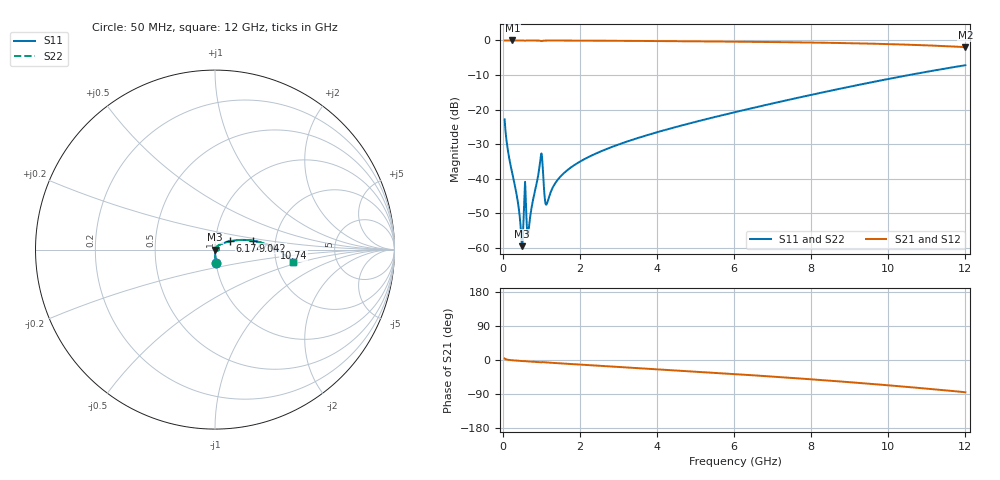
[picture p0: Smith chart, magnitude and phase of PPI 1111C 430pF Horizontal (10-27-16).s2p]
# MHz S MA R 50
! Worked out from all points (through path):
!   1601 points, 50 MHz to 12 GHz, reference 50 ohm
!   highest |S21| = 0.00 dB at 251.7 MHz (marker M1); lowest = -1.9 dB at 12 GHz (marker M2)
!   group delay of S21, straight-line fit = 19.3 ps
!   lowest |S11| = -59.5 dB at 505.6 MHz (marker M3), VSWR 1.00, Z = 50.1 - j0.027 ohm
!   |S11| at or under -10 dB: start of sweep to 10.54 GHz
!   |S22| runs from -59.5 to -7.2 dB; largest |S21 - S12| = 0
!   S11 on the Smith chart (normalised r, x): 50 MHz: 1.00, -0.14; 6.174 GHz: 1.18, +0.11; 9.042 GHz: 1.52, +0.16; 10.74 GHz: 1.99, +0.04; 12 GHz: 2.47, -0.42
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50  0.07214 -85.7  0.9968 3.9  0.9968 3.9  0.07214 -85.7
154.5625  0.02203 -88.5  0.9993 0.4  0.9993 0.4  0.02203 -88.5
251.6562  0.01174 -88.6  0.9995 -0.7  0.9995 -0.7  0.01174 -88.6
378.625  0.005193 -85.2  0.9994 -1.8  0.9994 -1.8  0.005193 -85.2
468.25  0.001946 -67.8  0.9992 -2.5  0.9992 -2.5  0.001946 -67.8
505.5938  0.001057 -14.7  0.9989 -2.8  0.9989 -2.8  0.001057 -14.7
587.75  0.007596 -28.0  0.9931 -3.1  0.9931 -3.1  0.007596 -28.0
684.8438  0.002063 43.7  0.9986 -3.9  0.9986 -3.9  0.002063 43.7
983.5938  0.02031 42.2  0.9864 -6.3  0.9864 -6.3  0.02031 42.2
1028.406  0.01797 -13.9  0.9822 -5.6  0.9822 -5.6  0.01797 -13.9
1110.562  0.004398 2.3  0.9956 -6.2  0.9956 -6.2  0.004398 2.3
1147.906  0.004374 29.1  0.9964 -6.5  0.9964 -6.5  0.004374 29.1
1469.062  0.01031 60.8  0.9963 -8.7  0.9963 -8.7  0.01031 60.8
2044.156  0.01819 58.2  0.9936 -12.3  0.9936 -12.3  0.01819 58.2
4038.312  0.0476 41.8  0.9797 -24.6  0.9797 -24.6  0.0476 41.8
6025  0.09177 29.8  0.9603 -37.2  0.9603 -37.2  0.09177 29.8
6174.375  0.09604 29.0  0.9586 -38.2  0.9586 -38.2  0.09604 29.0
8019.156  0.1641 19.2  0.9323 -51.1  0.9323 -51.1  0.1641 19.2
9042.375  0.2167 13.2  0.9115 -58.9  0.9115 -58.9  0.2167 13.2
10013.31  0.2781 6.8  0.8851 -66.9  0.8851 -66.9  0.2781 6.8
10737.78  0.3313 1.5  0.8596 -73.2  0.8596 -73.2  0.3313 1.5
12000  0.4377 -8.9  0.7999 -85.1  0.7999 -85.1  0.4377 -8.9
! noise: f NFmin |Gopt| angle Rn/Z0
50  0.0005222  0.9027  0.2994  0.001175
1372  0.006538  0.7991  7.589  0.00671
2701  0.01567  0.8336  14.86  0.01955
4031  0.0266  0.8546  22  0.03766
5360  0.03823  0.8677  28.95  0.05827
6682  0.05018  0.8772  35.63  0.0801
8012  0.06265  0.8855  42.09  0.1035
9341  0.07592  0.8934  48.28  0.1294
1.067e+04  0.09054  0.9016  54.17  0.1597
1.2e+04  0.1073  0.9101  59.78  0.1975
